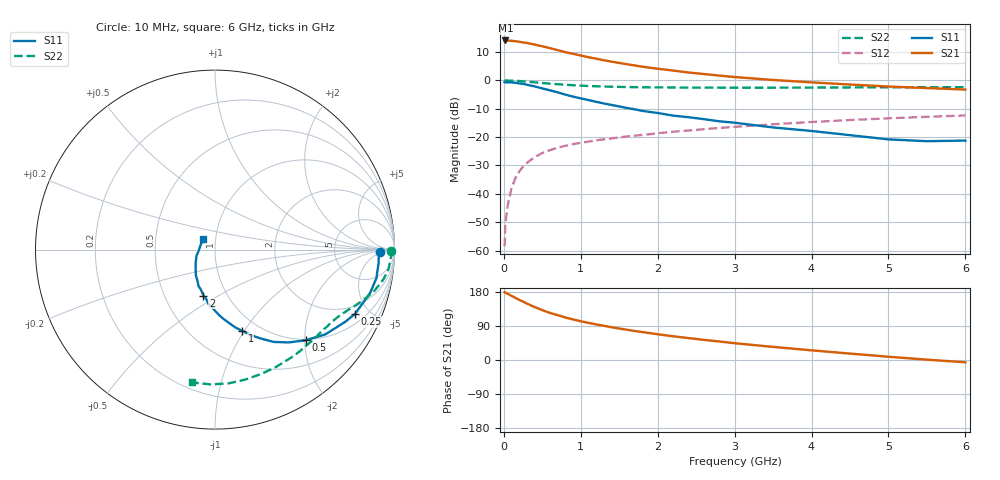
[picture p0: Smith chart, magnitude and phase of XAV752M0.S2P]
! SIEMENS Discrete & RF Semiconductors
! BFY180
! Si NPN RF Bipolar Junction Transistor in MICRO-X
! VCE = 0.75 V  IC = 2 mA
! Common Emitter S-Parameters:  May  1997
# GHz  S  MA  R  50
!  f  S11  S21  S12  S22
! GHz  MAG  ANG  MAG  ANG  MAG  ANG  MAG  ANG
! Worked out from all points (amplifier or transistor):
!   36 points, 10 MHz to 6 GHz, reference 50 ohm
!   highest |S21| = 14.0 dB at 20 MHz (marker M1)
!   |S21| within 3 dB of that: start of sweep to 641.2 MHz
!   unconditionally stable (mu >= 1): 1.213 GHz to end of sweep
!   at 250 MHz: K = 0.25, MSG = 21.8 dB, |S12| = -30.4 dB
!   at 1.4 GHz: K = 1.09, MAG = 11.7 dB, |S12| = -20.5 dB
!   at 6 GHz: K = 1.36, MAG = 1.0 dB, |S12| = -12.5 dB
!   S11 on the Smith chart (normalised r, x): 10 MHz: 23, -5; 250 MHz: 1.49, -4.05; 500 MHz: 0.98, -2.02; 1 GHz: 0.83, -0.98; 2 GHz: 0.78, -0.43; 6 GHz: 0.87, +0.10
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0.01  0.9209 -1.0  4.919 179.1  0.0012 84.3  0.9819 -0.3
0.02  0.9134 -1.9  4.986 177.7  0.003 88.4  0.985 -0.7
0.05  0.9145 -4.9  4.927 174.8  0.0062 83.8  0.9824 -2.1
0.1  0.913 -10.1  4.922 169.4  0.0125 85.2  0.9765 -4.2
0.2  0.8758 -19.9  4.731 158.7  0.0246 78.2  0.9635 -8.1
0.25  0.8583 -24.7  4.597 154.0  0.0301 74.4  0.953 -10.0
0.3  0.829 -29.1  4.499 148.9  0.0351 71.1  0.9403 -11.6
0.4  0.7755 -37.5  4.22 139.8  0.0442 66.4  0.9161 -14.6
0.5  0.7141 -45.0  3.939 131.5  0.0522 61.8  0.8896 -17.2
0.6  0.661 -51.5  3.647 124.2  0.0588 58.9  0.8662 -19.3
0.8  0.5551 -63.0  3.106 112.2  0.0698 54.2  0.8286 -22.9
1  0.4773 -71.6  2.709 102.2  0.0788 50.8  0.7997 -26.1
1.1  0.446 -75.6  2.529 98.1  0.0829 49.5  0.7883 -27.5
1.3  0.3886 -83.1  2.24 90.3  0.091 47.6  0.7721 -30.3
1.5  0.3445 -89.4  2.008 83.0  0.0981 45.9  0.7603 -33.3
2  0.2643 -104.1  1.587 67.9  0.1165 43.0  0.745 -40.5
2.2  0.2378 -109.1  1.473 62.6  0.1236 41.4  0.7414 -43.5
3  0.1781 -126.8  1.133 44.3  0.1507 36.2  0.7362 -55.0
3.5  0.1471 -137.1  1.006 34.6  0.1672 32.8  0.7367 -62.3
4.5  0.1076 -162.3  0.837 16.9  0.1985 24.6  0.7435 -76.9
5.5  0.0843 162.8  0.725 0.9  0.2267 15.9  0.7514 -92.1
6  0.0864 138.5  0.682 -6.0  0.2385 11.3  0.7508 -99.8
